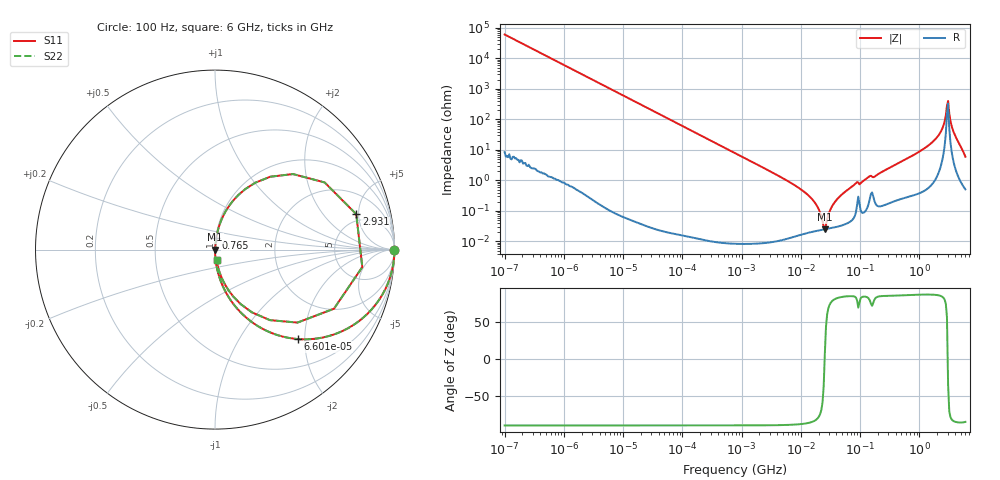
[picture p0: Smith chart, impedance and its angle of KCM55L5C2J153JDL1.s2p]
!Murata Part Number: KCM55L5C2J153JDL1
!These Parameters are Measured in Series Mode Connection
!Data Generated on Mar 13, 2026
!  o--ll--o
!Port1  Port2
!  o------o
!Operation Temp=25[degC], DC Bias Voltage=0[V]
!Freq. Start=100[Hz] Stop=6[GHz] 401[Steps]
# Hz S RI R 50
!Freq.(Hz) S11(Real) S11(Imag) S21(Real) S21(Imag) S12(Real) S12(Imag) S22(Real) S22(Imag)
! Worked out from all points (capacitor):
!   401 points, 100 Hz to 6 GHz, reference 50 ohm
!   read as one part in series: C = 26 nF near 109 Hz
!   lowest |Z| = 25.1 mohm at 25.46 MHz (marker M1)
!   series resonance near 25.27 MHz, so ESL is about 1.5 nH
!   S11 on the Smith chart (normalised r, x): 100 Hz: open; 66 kHz: 1.00, -1.85; 765 MHz: 1.01, +0.13; 2.931 GHz: 4.05, +4.68; 6 GHz: 1.01, -0.12
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100  1 -0.00164  2.9e-06 0.00164  2.9e-06 0.00164  1 -0.00164
2008  0.9989 -0.0328  0.00108 0.0328  0.00108 0.0328  0.9989 -0.0328
14402  0.9475 -0.223  0.0525 0.223  0.0525 0.223  0.9475 -0.223
40335  0.697 -0.4595  0.303 0.4595  0.303 0.4595  0.697 -0.4595
66005  0.4621 -0.4985  0.5379 0.4985  0.5379 0.4985  0.4621 -0.4985
176758  0.1071 -0.309  0.8929 0.309  0.8929 0.309  0.1071 -0.309
774597  0.00627 -0.0784  0.9937 0.0784  0.9937 0.0784  0.00627 -0.0784
6644369  0.000202 -0.00851  0.9998 0.00851  0.9998 0.00851  0.000202 -0.00851
1.555665e7  0.000211 -0.0024  0.9998 0.0024  0.9998 0.0024  0.000211 -0.0024
2.545746e7  0.000248 3.49e-05  0.9998 -3.49e-05  0.9998 -3.49e-05  0.000248 3.49e-05
3.482834e7  0.000282 0.00155  0.9997 -0.00155  0.9997 -0.00155  0.000282 0.00155
4.983056e7  0.000348 0.0035  0.9997 -0.0035  0.9997 -0.0035  0.000348 0.0035
8.527865e7  0.000968 0.00801  0.999 -0.00801  0.999 -0.00801  0.000968 0.00801
3.124326e8  0.00244 0.0255  0.9976 -0.0255  0.9976 -0.0255  0.00244 0.0255
7.650043e8  0.00726 0.0639  0.9927 -0.0639  0.9927 -0.0639  0.00726 0.0639
2.048624e9  0.0835 0.2505  0.9165 -0.2505  0.9165 -0.2505  0.0835 0.2505
2.562649e9  0.3082 0.4061  0.6918 -0.4061  0.6918 -0.4061  0.3082 0.4061
2.931063e9  0.7871 0.1974  0.2129 -0.1974  0.2129 -0.1974  0.7871 0.1974
3.205649e9  0.6629 -0.3293  0.3371 0.3293  0.3371 0.3293  0.6629 -0.3293
3.505958e9  0.3058 -0.3929  0.6942 0.3929  0.6942 0.3929  0.3058 -0.3929
4.193612e9  0.074 -0.2246  0.926 0.2246  0.926 0.2246  0.074 -0.2246
6e9  0.00854 -0.0589  0.9915 0.0589  0.9915 0.0589  0.00854 -0.0589
